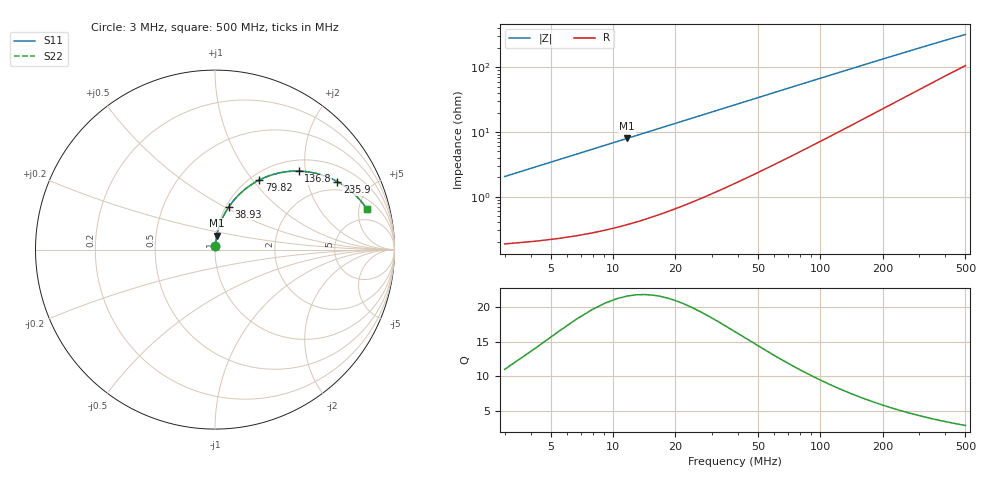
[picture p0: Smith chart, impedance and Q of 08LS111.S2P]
! Coilcraft 0805LS-111 Chip Inductor
! 18 September 2002
# MHZ S MA R 50
!Freq  MagS11  AngS11  MagS21  AngS21  MagS12  AngS12  MagS22  AngS22
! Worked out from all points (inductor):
!   403 points, 3 MHz to 500 MHz, reference 50 ohm
!   read as one part in series: L = 108 nH near 5.478 MHz
!   highest Q = 21.6 at 11.67 MHz (marker M1), where L = 108 nH
!   S11 on the Smith chart (normalised r, x): 3 MHz: 1.00, +0.04; 38.93 MHz: 1.03, +0.53; 79.82 MHz: 1.10, +1.08; 136.8 MHz: 1.24, +1.84; 235.9 MHz: 1.60, +3.10; 500 MHz: 3.12, +6.08
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3  0.0204 83.6  0.9979 -1.2  0.9979 -1.2  0.0204 83.6
4.239  0.02877 84.3  0.9975 -1.6  0.9975 -1.6  0.02877 84.3
6.717  0.04552 84.3  0.9965 -2.6  0.9965 -2.6  0.04552 84.3
7.956  0.05389 84.0  0.9958 -3.1  0.9958 -3.1  0.05389 84.0
11.673  0.0789 82.8  0.9932 -4.5  0.9932 -4.5  0.0789 82.8
16.629  0.1119 80.9  0.9885 -6.4  0.9885 -6.4  0.1119 80.9
22.824  0.1525 78.4  0.9808 -8.8  0.9808 -8.8  0.1525 78.4
30.258  0.1997 75.4  0.969 -11.5  0.969 -11.5  0.1997 75.4
38.931  0.2524 71.9  0.9524 -14.6  0.9524 -14.6  0.2524 71.9
47.604  0.3023 68.6  0.933 -17.6  0.933 -17.6  0.3023 68.6
57.516  0.3555 64.9  0.9084 -20.8  0.9084 -20.8  0.3555 64.9
79.818  0.4594 57.5  0.8472 -27.2  0.8472 -27.2  0.4594 57.5
86.013  0.4846 55.7  0.8296 -28.8  0.8296 -28.8  0.4846 55.7
109.554  0.5666 49.3  0.7629 -34.3  0.7629 -34.3  0.5666 49.3
136.812  0.639 43.2  0.6905 -39.3  0.6905 -39.3  0.639 43.2
169.026  0.7011 37.4  0.615 -43.9  0.615 -43.9  0.7011 37.4
201.24  0.7456 32.9  0.5512 -47.3  0.5512 -47.3  0.7456 32.9
235.932  0.7802 29.0  0.4938 -50.0  0.4938 -50.0  0.7802 29.0
252.039  0.7929 27.5  0.4707 -51.0  0.4707 -51.0  0.7929 27.5
335.052  0.8372 21.5  0.378 -54.2  0.378 -54.2  0.8372 21.5
418.065  0.8617 17.6  0.3157 -55.6  0.3157 -55.6  0.8617 17.6
500  0.8766 14.9  0.2722 -55.8  0.2722 -55.8  0.8766 14.9
